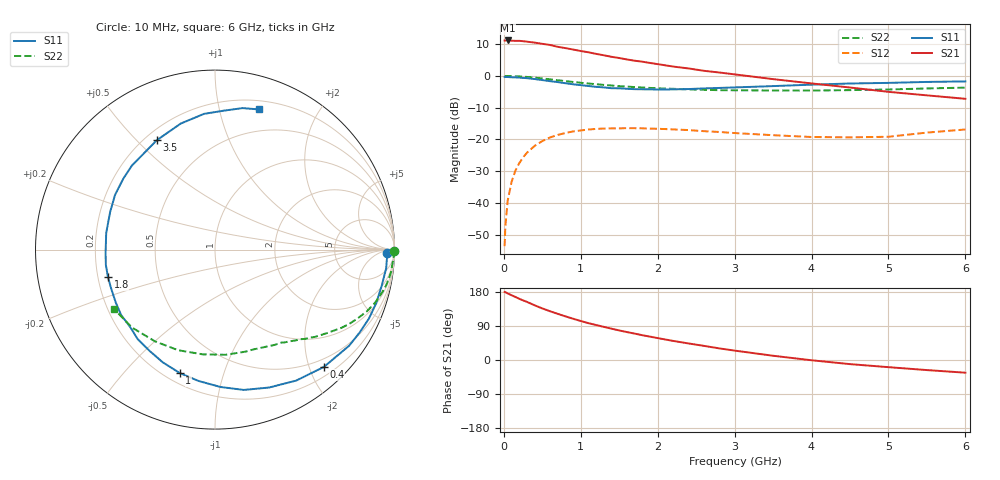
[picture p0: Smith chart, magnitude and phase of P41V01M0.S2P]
! SIEMENS Small Signal Semiconductors
! BFP182
! Si NPN RF Bipolar Junction Transistor in SOT143
! VCE = 1 V  IC = 1 mA
! Common Emitter S-Parameters:  March  1996
# GHz  S  MA  R  50
!  f  S11  S21  S12  S22
! GHz  MAG  ANG  MAG  ANG  MAG  ANG  MAG  ANG
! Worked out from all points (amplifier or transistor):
!   36 points, 10 MHz to 6 GHz, reference 50 ohm
!   highest |S21| = 11.1 dB at 50 MHz (marker M1)
!   |S21| within 3 dB of that: start of sweep to 931.7 MHz
!   unconditionally stable (mu >= 1): 2.544 GHz to end of sweep
!   at 250 MHz: K = 0.10, MSG = 18.3 dB, |S12| = -25.6 dB
!   at 1.4 GHz: K = 0.56, MSG = 11.3 dB, |S12| = -16.5 dB
!   at 6 GHz: K = 1.21, MAG = 2.0 dB, |S12| = -16.9 dB
!   S11 on the Smith chart (normalised r, x): 10 MHz: 39, -20; 400 MHz: 0.35, -2.25; 1 GHz: 0.26, -0.72; 1.8 GHz: 0.24, -0.12; 3.5 GHz: 0.25, +0.57; 6 GHz: 0.28, +1.32
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0.01  0.9607 -1.2  3.597 179.5  0.0021 86.1  0.9974 -0.5
0.02  0.9594 -2.6  3.593 178.9  0.0043 87.6  0.9912 -0.9
0.05  0.9594 -6.2  3.605 175.6  0.0109 88.3  0.9964 -2.4
0.1  0.9508 -12.0  3.584 170.9  0.0214 81.2  0.9908 -4.9
0.15  0.9466 -18.3  3.549 166.4  0.0323 78.4  0.989 -7.3
0.25  0.9289 -29.8  3.51 157.3  0.0522 71.4  0.9732 -12.0
0.4  0.8919 -47.1  3.334 144.3  0.0793 60.8  0.9394 -18.4
0.5  0.8587 -58.2  3.192 136.1  0.0943 54.4  0.9118 -22.3
0.6  0.8254 -68.6  3.063 128.7  0.1075 48.2  0.882 -25.8
0.8  0.7661 -87.7  2.734 115.2  0.1263 37.9  0.8278 -31.8
1  0.7153 -105.9  2.458 102.9  0.1386 29.2  0.7792 -36.6
1.1  0.6924 -114.8  2.349 97.2  0.1433 25.4  0.758 -38.9
1.4  0.6396 -137.8  1.995 82.6  0.1496 15.2  0.7059 -44.8
1.6  0.6264 -152.1  1.813 73.7  0.1507 10.1  0.6792 -48.0
1.8  0.6156 -165.7  1.671 65.4  0.1499 6.2  0.6568 -51.2
2.2  0.6132 171.3  1.402 50.4  0.144 -1.1  0.6263 -58.0
2.8  0.6459 142.3  1.13 30.7  0.1312 -7.0  0.5959 -69.0
3.5  0.6904 118.0  0.889 11.2  0.1168 -8.7  0.589 -84.2
4  0.7278 105.2  0.761 -0.7  0.1094 -5.0  0.5876 -96.7
4.5  0.7588 94.6  0.656 -10.9  0.108 -0.9  0.5969 -110.0
5.5  0.8031 79.0  0.494 -26.6  0.1283 8.7  0.6343 -136.8
6  0.8184 72.6  0.436 -33.5  0.1436 8.2  0.6535 -149.8
